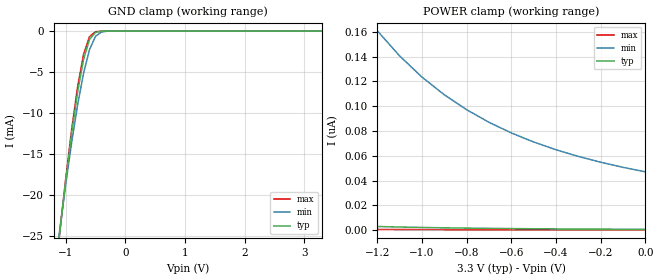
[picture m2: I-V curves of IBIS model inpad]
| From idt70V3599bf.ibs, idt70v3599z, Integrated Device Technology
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|   Model inpad
[Model]   inpad
Model_type   Input
Vinl =  0.80000V
Vinh =  2.00000V
C_comp   4.50000pF   NA   NA
[Temperature Range]   25.00000   100.00000   0.000
[Voltage Range]   3.30000V   3.15000V   3.45000V
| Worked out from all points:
|   GND clamp passes 1 mA (typ) near -0.60 V on its own axis
[GND_clamp]
| voltage   I(typ)   I(min)   I(max)
-3.3V     -188.6mA   -176.3mA   -192.8mA
-1.1V     -24.44mA   -24.14mA   -24.52mA
-1V       -18.16mA   -18.62mA   -17.94mA
-900mV    -12.39mA   -13.52mA   -11.92mA
-800mV    -7.362mA   -8.949mA   -6.715mA
-700mV    -3.406mA   -5.088mA   -2.784mA
-600mV    -997.5uA   -2.222mA   -658.4uA
-500mV    -153.8uA   -629.2uA   -78.71uA
-400mV    -14.38uA   -107.8uA   -5.649uA
-300mV    -881nA     -13.18uA   -246.3nA
3.3V      614.3pA    52.62nA    78.77pA
[POWER_clamp]
| voltage   I(typ)   I(min)   I(max)
-3.3V     101.8nA    3.951uA    22.06nA
-3.1V     74.02nA    2.958uA    15.9nA
-2.9V     53.46nA    2.199uA    11.36nA
-2.7V     38.34nA    1.624uA    8.071nA
-2.5V     27.33nA    1.192uA    5.695nA
-2V       11.47nA    541.3nA    2.317nA
-1.2V     2.895nA    160.9nA    540pA
-1V       2.108nA    123.5nA    389.4pA
-900mV    1.815nA    109.2nA    323.4pA
-700mV    1.372nA    86.98nA    238pA
-400mV    942.1pA    64.82nA    157pA
0V        614.3pA    46.98nA    89.71pA
